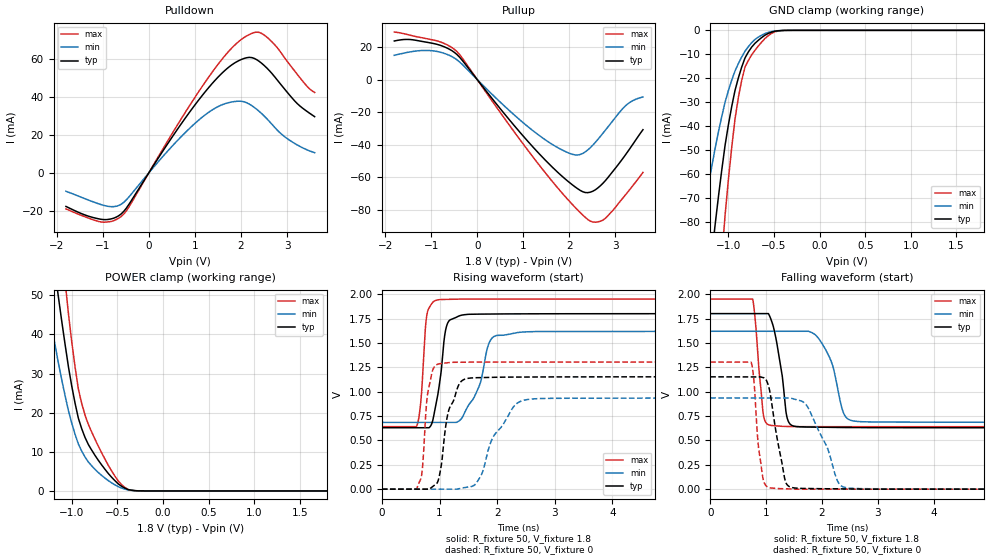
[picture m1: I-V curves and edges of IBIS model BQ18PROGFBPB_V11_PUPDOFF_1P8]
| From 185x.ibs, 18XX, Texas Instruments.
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|   Model Cell BQ18PROGFBPB_V11_PUPDOFF_1P8
|BQ18PROGFBPB_V11_PUPDOFF_1P8
[Model]   BQ18PROGFBPB_V11_PUPDOFF_1P8
Model_type   I/O
Polarity   Non-Inverting
Enable   Active-Low
Vinl =  0.63
Vinh =  1.17
Cref =  15pF
Rref =  100.0000M
Vref =  0V
Vmeas =  0.9
C_comp   2.023746p   1.863846p   2.096173p
[Model Spec]
Vinl   0.63   0.567   0.6825
Vinh   1.17   1.053   1.2675
[Temperature Range]   25   125   -40
[Voltage Range]   1.8   1.62   1.95
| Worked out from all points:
|   slope of the pulldown table from 0 to 0.27 V, typ, clamps not added: 26.3 ohm
|   slope of the pullup table from 0 to 0.27 V, typ, clamps not added: 27.7 ohm
|   GND clamp passes 1 mA (typ) near -0.54 V on its own axis
|   POWER clamp passes 1 mA (typ) near -0.44 V on its own axis
|   rising waveform, R_fixture 50, V_fixture 1.8: 20-80 % time 151ps typ, 309ps min, 83.7ps max; typ from 0.63 V to 1.8 V
|   rising waveform, R_fixture 50, V_fixture 0: 20-80 % time 225ps typ, 434ps min, 105ps max; typ from 0 V to 1.15 V
|   falling waveform, R_fixture 50, V_fixture 1.8: 20-80 % time 171ps typ, 275ps min, 111ps max; typ from 1.8 V to 0.63 V
|   falling waveform, R_fixture 50, V_fixture 0: 20-80 % time 205ps typ, 392ps min, 115ps max; typ from 1.15 V to 0 V
| Nom Voltages:
|   BIASFET=1.8, VBBNW=1.1, VDD=1.1, VDDS=1.8, VSS=0, VSSS=0
| Min Voltages:
|   BIASFET=1.62, VBBNW=0.99, VDD=0.99, VDDS=1.62, VSS=0, VSSS=0
| Max Voltages:
|   BIASFET=1.95, VBBNW=1.21, VDD=1.21, VDDS=1.95, VSS=0, VSSS=0
[POWER_clamp]
|   voltage   I(typ)   I(min)   I(max)
-1.8V     178.9mA    128mA      243.2mA
-1.291V   75.76mA    51.65mA    107.4mA
-1.255V   68.98mA    46.64mA    97.96mA
-1.145V   49.38mA    32.55mA    70.53mA
-1.073V   37.35mA    24.29mA    53.42mA
-1.036V   31.7mA     20.49mA    45.27mA
-963.6mV  22.39mA    14.45mA    31.64mA
-890.9mV  15.9mA     10.19mA    22.36mA
-781.8mV  10.44mA    6.418mA    15.08mA
-527.3mV  2.627mA    1.561mA    3.8mA
-309.1mV  78.64uA    63.19uA    57.71uA
1.8V      -4.158nA   -210nA     -5.748nA
[Pulldown]
|   voltage   I(typ)   I(min)   I(max)
-1.8V     -17.77mA   -9.748mA   -19.05mA
-1.036V   -24.56mA   -16.8mA    -25.99mA
-763.6mV  -23.98mA   -17.86mA   -25.3mA
-545.5mV  -20.4mA    -15.61mA   -21.81mA
545.5mV   20.33mA    15.12mA    22.33mA
1.2V      42.13mA    30.21mA    47.14mA
1.745V    56.06mA    37.17mA    64.53mA
2.182V    61.03mA    36.32mA    73.12mA
2.4V      58.85mA    32.4mA     74.19mA
2.564V    55.36mA    28.55mA    71.7mA
3V        42.72mA    18.17mA    59.07mA
3.6V      29.69mA    10.66mA    42.5mA
[Pullup]
|   voltage   I(typ)   I(min)   I(max)
-1.8V     23.69mA    14.89mA    29.16mA
-1.036V   22.62mA    17.82mA    24.76mA
-709.1mV  20.05mA    16.02mA    22.07mA
-436.4mV  15.28mA    12.07mA    17.09mA
600mV     -21.35mA   -16.51mA   -24.17mA
1.309V    -44.48mA   -33.57mA   -51.19mA
1.964V    -62.36mA   -44.86mA   -73.59mA
2.291V    -68.93mA   -45.43mA   -83.23mA
2.509V    -68.65mA   -40.36mA   -87.54mA
2.727V    -63.85mA   -33.1mA    -86.46mA
3.218V    -46.34mA   -16.18mA   -70.92mA
3.6V      -30.82mA   -10.7mA    -57.09mA
[GND_clamp]
|   voltage   I(typ)   I(min)   I(max)
-1.8V     -337.7mA   -206.7mA   -550.8mA
-1.291V   -133.7mA   -80.77mA   -221.4mA
-1.145V   -81.03mA   -49.16mA   -133.6mA
-1.073V   -58.22mA   -35.89mA   -94.75mA
-1.036V   -47.89mA   -29.95mA   -77.04mA
-927.3mV  -25.01mA   -16.92mA   -36.88mA
-854.5mV  -15.35mA   -11.15mA   -20.84mA
-781.8mV  -9.051mA   -6.811mA   -12.6mA
-636.4mV  -3.048mA   -2.032mA   -4.945mA
-490.9mV  -357.6uA   -261.1uA   -600.3uA
-381.8mV  -30.89uA   -27.8uA    -45.52uA
1.8V      460.3pA    2.186uA    3.34nA
[Ramp]
| variable   typ   min   max
dV/dt_f 0.71599785/0.17671718n 0.57199675/0.28732029n 0.80224867/0.11416901n
dV/dt_r 0.69348718/0.22552866n 0.56299525/0.43464041n 0.78654679/0.105397n
R_load = 50
[Rising Waveform]
R_fixture = 50
V_fixture = 1.8
V_fixture_min = 1.62
V_fixture_max = 1.95
|   time   V(typ)   V(min)   V(max)
0s        630.3mV    684.7mV    641.1mV
604.3ps   630.3mV    684.7mV    646.1mV
677.1ps   630.3mV    684.7mV    905.9mV
780ps     630.3mV    684.7mV    1.785V
966.8ps   956.9mV    684.7mV    1.941V
1.157ns   1.721V     684.7mV    1.948V
1.594ns   1.795V     935.5mV    1.95V
1.852ns   1.796V     1.488V     1.95V
2.003ns   1.797V     1.577V     1.95V
11.2ns    1.8V       1.62V      1.95V
[Rising Waveform]
R_fixture = 50
V_fixture = 0
V_fixture_min = 0
V_fixture_max = 0
|   time   V(typ)   V(min)   V(max)
0s        0V         0V         0V
607.9ps   0V         0V         8.921mV
694.7ps   0V         0V         163.6mV
801.7ps   0V         0V         1.006V
1.003ns   152.3mV    0V         1.287V
1.161ns   810.3mV    0V         1.299V
1.494ns   1.137V     21.67mV    1.303V
1.952ns   1.147V     556.2mV    1.303V
2.514ns   1.151V     918.5mV    1.304V
11.2ns    1.153V     936.1mV    1.304V
[Falling Waveform]
R_fixture = 50
V_fixture = 1.8
V_fixture_min = 1.62
V_fixture_max = 1.95
|   time   V(typ)   V(min)   V(max)
0s        1.8V       1.619V     1.95V
760.7ps   1.8V       1.619V     1.95V
945ps     1.8V       1.619V     788.7mV
1.072ns   1.765V     1.619V     655.5mV
1.37ns    749.5mV    1.619V     643mV
1.514ns   644.2mV    1.619V     641.6mV
1.978ns   635.8mV    1.515V     640.7mV
2.386ns   632.2mV    781.8mV    640.6mV
2.566ns   631.6mV    699.4mV    640.6mV
11.2ns    629.7mV    684.6mV    640.3mV
[Falling Waveform]
R_fixture = 50
V_fixture = 0
V_fixture_min = 0
V_fixture_max = 0
|   time   V(typ)   V(min)   V(max)
0s        1.152V     935.6mV    1.303V
735.9ps   1.152V     935.6mV    1.296V
930.7ps   1.147V     935.6mV    156.7mV
1.066ns   1.006V     935.6mV    14.1mV
1.334ns   107.3mV    935.6mV    3.743mV
1.48ns    14.54mV    928.1mV    2.188mV
1.745ns   6.747mV    843.2mV    0V
2.281ns   3.16mV     81.55mV    0V
2.443ns   2.599mV    13.96mV    0V
11.2ns    0V         0V         0V
